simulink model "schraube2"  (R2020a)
settings: Solver=VariableStepDiscrete  StartTime=0.0  StopTime=30  MaxStep=0.1  RelTol=1e-3  EnableMultiTasking=on
libraries: simulink x1

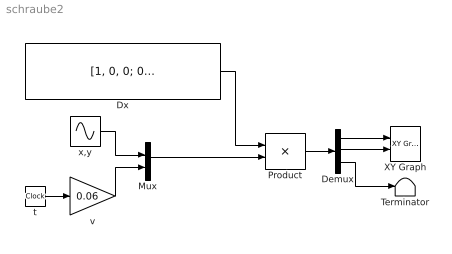
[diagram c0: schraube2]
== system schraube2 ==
  Demux : Demux  Outputs=3
  Dx : Constant  Value=[1, 0, 0; 0, cos(pi/6), -sin(pi/6); 0, sin(pi/6), cos(pi/6)]
  Mux : Mux  Inputs=2
  Product : Product  Multiplication=Matrix(*)  RndMeth=Zero
  Terminator : Terminator
  XY Graph : simulink/Sinks/XY Graph  xmin=-1.2  xmax=1.2  ymin=-3  ymax=2  st=-1
  t : Clock
  v : Gain  Gain=0.06
  x,y : Sin  Amplitude=[1,1]  Frequency=[1, 1]  Phase=[-pi/2, 0]  SampleTime=0
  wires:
  t/1 -> v/1
  x,y/1 -> Mux/1
  v/1 -> Mux/2
  Mux/1 -> Product/2
  Dx/1 -> Product/1
  Product/1 -> Demux/1
  Demux/1 -> XY Graph/1
  Demux/2 -> XY Graph/2
  Demux/3 -> Terminator/1
